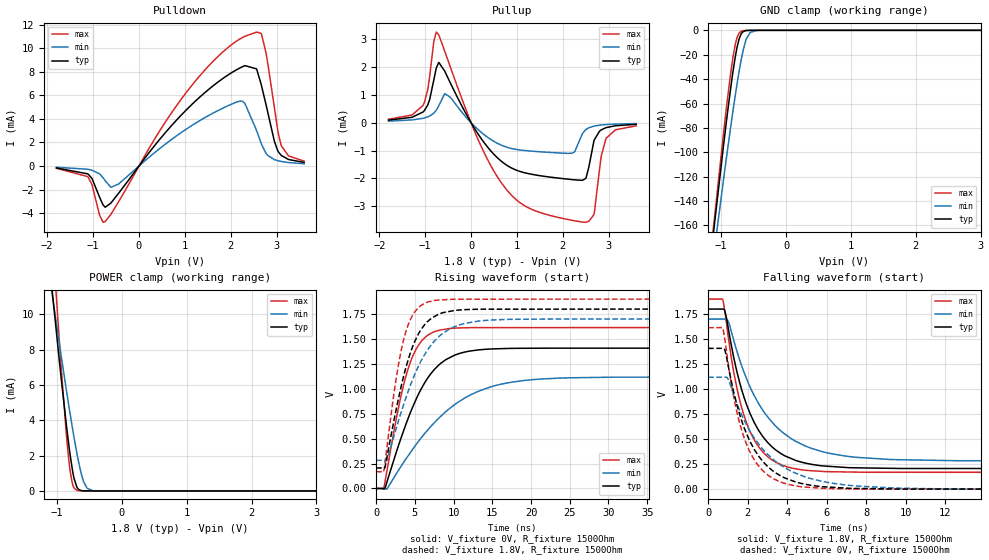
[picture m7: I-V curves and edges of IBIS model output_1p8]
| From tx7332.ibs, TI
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|   output_1p8 Model
[Model]   output_1p8
Model_type   3-state
Polarity   Non-Inverting
Vmeas = 0.9
Vref = 0
Cref = 2pF
Rref = 100000
|   typ   min   max
C_comp   6.133pF   6.021pF   6.247pF
| Where Nom  PVT is Nominal Process, 1.8V, 27C
|   Fast PVT is Strong Process,  1.9V, 0C
|   Slow PVT is Weak Process,   1.7V, 100C
[Voltage Range]   1.8   1.7   1.9
|Junction Temperature
[Temperature Range]   27   100   0
[Pullup Reference]   1.8   1.7   1.9
[Pulldown Reference]   0   0   0
[Power Clamp Reference]   1.8   1.7   1.9
[GND Clamp Reference]   0   0   0
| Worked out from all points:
|   slope of the pulldown table from 0 to 0.27 V, typ, clamps not added: 195 ohm
|   slope of the pullup table from 0 to 0.27 V, typ, clamps not added: 397 ohm
|   GND clamp passes 1 mA (typ) near -0.66 V on its own axis
|   POWER clamp passes 1 mA (typ) near -0.75 V on its own axis
|   falling waveform, V_fixture 1.8V, R_fixture 1500Ohm: 20-80 % time 1.64ns typ, 2.38ns min, 1.28ns max; typ from 1.8 V to 0.206 V
|   rising waveform, V_fixture 0V, R_fixture 1500Ohm: 20-80 % time 4.55ns typ, 7.95ns min, 2.81ns max; typ from 0 V to 1.41 V
|   rising waveform, V_fixture 1.8V, R_fixture 1500Ohm: 20-80 % time 3.12ns typ, 4.43ns min, 2.21ns max; typ from 0.206 V to 1.8 V
|   falling waveform, V_fixture 0V, R_fixture 1500Ohm: 20-80 % time 1.63ns typ, 2.42ns min, 1.26ns max; typ from 1.41 V to 0 V
[Pulldown]
|   Voltage   I(typ)   I(min)   I(max)
-1.8V     -163uA     -100.7uA   -192.2uA
-1.12V    -657.8uA   -271.7uA   -891.6uA
-736.2mV  -3.493mA   -1.242mA   -4.709mA
-444.6mV  -2.307mA   -1.523mA   -3.031mA
916.2mV   4.297mA    2.824mA    5.642mA
2.126V    8.158mA    5.417mA    10.59mA
2.309V    8.514mA    5.313mA    11mA
2.569V    8.186mA    2.969mA    11.36mA
2.768V    5.241mA    1.085mA    9.638mA
2.952V    2.111mA    547.3uA    4.983mA
3.103V    900.9uA    386.9uA    1.728mA
3.6V      306.6uA    195.6uA    415.6uA
[GND Clamp]
|   Voltage   I(typ)   I(min)   I(max)
-1.8V     -499mA     -477.9mA   -522.9mA
-1.13V    -171.5mA   -190.7mA   -167.5mA
-963mV    -94.09mA   -122.1mA   -84.02mA
-898.2mV  -65.85mA   -96.5mA    -54.13mA
-833.4mV  -39.66mA   -71.79mA   -27.58mA
-774mV    -19.23mA   -50.38mA   -9.642mA
-725.4mV  -7.453mA   -34.29mA   -2.488mA
-693mV    -3.082mA   -24.66mA   -869.5uA
-612mV    -190.2uA   -7.045mA   -83.45uA
-552.6mV  -21.63uA   -1.699mA   -16.88uA
-444.6mV  -370nA     -74.56uA   -631.6nA
3.6V      0A         0A         0A
[Pullup]
|   Voltage   I(typ)   I(min)   I(max)
-1.8V     92.06uA    55.05uA    122.9uA
-1.049V   382uA      156.6uA    615.1uA
-757.8mV  1.965mA    448uA      3.25mA
-574.2mV  1.85mA     1.041mA    2.566mA
160.2mV   -422.6uA   -255.6uA   -629.7uA
765mV     -1.511mA   -871.6uA   -2.383mA
2.201V    -2.04mA    -1.094mA   -3.501mA
2.428V    -2.068mA   -393.3uA   -3.566mA
2.677V    -673.7uA   -123.4uA   -3.306mA
2.839V    -257.7uA   -81.99uA   -1.197mA
2.947V    -176.5uA   -66.66uA   -554.9uA
3.6V      -58.02uA   -30.49uA   -111.8uA
[POWER Clamp]
|   Voltage   I(typ)   I(min)   I(max)
-1.8V     38.72mA    29.91mA    56.93mA
-1.082V   11.59mA    11.31mA    14.93mA
-963mV    7.329mA    8.329mA    8.429mA
-855mV    3.718mA    5.7mA      3.175mA
-817.2mV  2.584mA    4.811mA    1.725mA
-795.6mV  1.99mA     4.314mA    1.076mA
-752.4mV  987.9uA    3.35mA     293.9uA
-693mV    210.7uA    2.12mA     28.25uA
-590.4mV  4.841uA    527.8uA    341.1nA
-536.4mV  577.9nA    150.7uA    9.467nA
-444.6mV  0A         10.14uA    0A
3.6V      0A         0A         0A
[Ramp]
R_load = 1500
|   typ   min   max
dV/dt_r   0.844441/4.55671e-09   0.670885/7.93994e-09   0.9686/2.81633e-09
dV/dt_f   0.95665/1.64124e-09   0.850728/2.38219e-09   1.03913/1.27876e-09
[Falling Waveform]
V_fixture = 1.8V
V_fixture_min = 1.7V
V_fixture_max = 1.9V
R_fixture = 1500Ohm
C_fixture = 0F
|   Time   V(typ)   V(min)   V(max)
0s        1.8V       1.7V       1.9V
748ps     1.8V       1.7V       1.888V
986ps     1.642V     1.69V      1.566V
1.456ns   1.173V     1.379V     1.006V
2.245ns   702.4mV    969.3mV    523.8mV
3.24ns    421.3mV    669.4mV    291.1mV
4.575ns   278.3mV    464.5mV    198.2mV
6.306ns   225.8mV    351.5mV    174.1mV
9.265ns   208.2mV    295.9mV    168.8mV
50ns      205.6mV    282.1mV    168.1mV
[Rising Waveform]
V_fixture = 0V
V_fixture_min = 0V
V_fixture_max = 0V
R_fixture = 1500Ohm
C_fixture = 0F
|   Time   V(typ)   V(min)   V(max)
0s        -47.13nV   -10.01nV   -1.817nV
1.052ns   -2.919mV   -1.085mV   23.03mV
1.401ns   65.21mV    -4.798mV   177.8mV
3.033ns   463.4mV    199.5mV    864mV
4.372ns   750.6mV    354.3mV    1.257V
5.706ns   981.8mV    496.8mV    1.464V
7.38ns    1.181V     648.7mV    1.568V
11.04ns   1.361V     887.6mV    1.611V
17.59ns   1.405V     1.067V     1.614V
50ns      1.407V     1.118V     1.614V
[Rising Waveform]
V_fixture = 1.8V
V_fixture_min = 1.7V
V_fixture_max = 1.9V
R_fixture = 1500Ohm
C_fixture = 0F
|   Time   V(typ)   V(min)   V(max)
0s        205.6mV    282.1mV    168.1mV
1.047ns   201.5mV    281.1mV    192.5mV
1.381ns   307mV      282mV      399.1mV
2.613ns   800.8mV    607.6mV    1.113V
3.775ns   1.193V     892.7mV    1.555V
4.782ns   1.436V     1.106V     1.747V
6.209ns   1.637V     1.336V     1.855V
9.265ns   1.773V     1.59V      1.895V
13.67ns   1.798V     1.683V     1.899V
50ns      1.8V       1.7V       1.9V
[Falling Waveform]
|Gnd
V_fixture = 0V
V_fixture_min = 0V
V_fixture_max = 0V
R_fixture = 1500Ohm
C_fixture = 0F
|   Time   V(typ)   V(min)   V(max)
0s        1.407V     1.118V     1.614V
740ps     1.408V     1.119V     1.608V
968.2ps   1.28V      1.115V     1.319V
1.456ns   840.6mV    857.7mV    766.3mV
2.245ns   429.4mV    537.5mV    322.4mV
3.033ns   222.6mV    342.6mV    138.6mV
4.372ns   76.13mV    164.2mV    34.18mV
6.895ns   11.43mV    43.42mV    3.945mV
11.04ns   1.016mV    5.11mV     664.4uV
50ns      -18.69nV   -8.639nV   -36.31nV
